PROGRAM MAIN
VAR
	{attribute 'OPC.UA.DA' := '1'}
	{attribute 'OPC.UA.DA.StructuredType' :='1'}
	structure_test	:ST_test;//结构体
	
	{attribute 'OPC.UA.DA' :='1'}
	iteration3 		:INT;//整数
	{attribute 'OPC.UA.DA' :='1'}
	iter2			:INT;//整数
	{attribute 'OPC.UA.DA' := '1'}
	i			: 	INT := 0;
END_VAR

structure_test.a		:= structure_test.a + 1;
iteration3				:= iteration3 + 1; 
iter2					:= iter2 + 2;

END_PROGRAM
